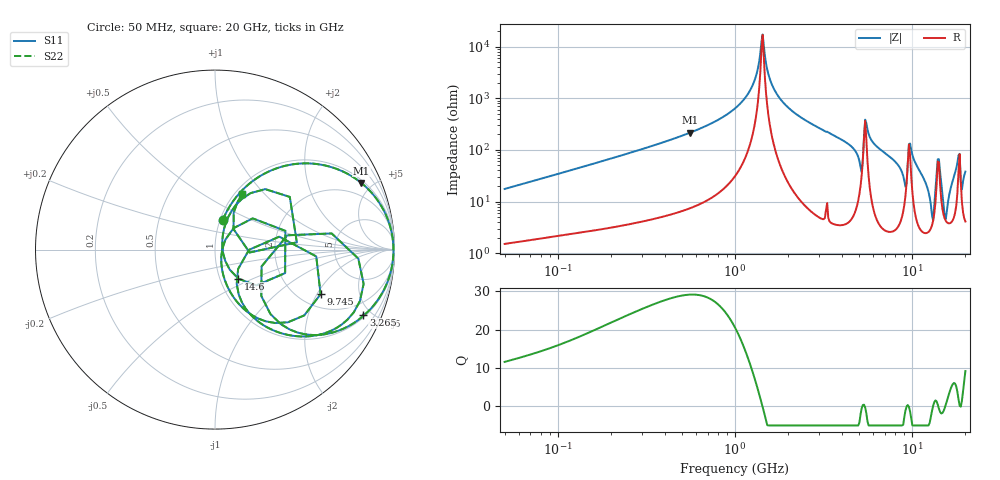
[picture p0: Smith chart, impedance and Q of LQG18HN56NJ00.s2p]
!Murata Part Number: LQG18HN56NJ00
!These Parameters are Measured in Series Mode Connection
!  o--[Z]--o
!Port1  Port2
!  o-------o
!Freq. Start=50[MHz] Stop=20[GHz], 401[Steps]
# Hz S RI R 50
!Freq.(Hz) S11(Real) S11(Imag) S21(Real) S21(Imag) S12(Real) S12(Imag) S22(Real) S22(Imag)
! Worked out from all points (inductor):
!   401 points, 50 MHz to 20 GHz, reference 50 ohm
!   read as one part in series: L = 54.9 nH near 51.52 MHz
!   highest Q = 29.1 at 557.6 MHz (marker M1), where L = 61.5 nH
!   self-resonance near 1.411 GHz
!   S11 on the Smith chart (normalised r, x): 50 MHz: 1.03, +0.35; 3.265 GHz: 1.14, -4.47; 9.745 GHz: 2.56, -2.15; 14.6 GHz: 1.22, -0.41; 20 GHz: 1.08, +0.76
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5e7  0.0431 0.1644  0.9569 -0.1644  0.9569 -0.1644  0.0431 0.1644
1.364002e8  0.1904 0.3664  0.8096 -0.3664  0.8096 -0.3664  0.1904 0.3664
3.721004e8  0.6303 0.4646  0.3697 -0.4646  0.3697 -0.4646  0.6303 0.4646
5.575697e8  0.8149 0.3716  0.1851 -0.3716  0.1851 -0.3716  0.8149 0.3716
1e9  0.9688 0.1511  0.0312 -0.1511  0.0312 -0.1511  0.9688 0.1511
1.251922e9  0.9906 0.0566  0.00943 -0.0566  0.00943 -0.0566  0.9906 0.0566
1.432596e9  0.9943 -0.00107  0.00567 0.00107  0.00567 0.00107  0.9943 -0.00107
1.740566e9  0.9873 -0.0856  0.0127 0.0856  0.0127 0.0856  0.9873 -0.0856
2.728004e9  0.9036 -0.2855  0.0964 0.2855  0.0964 0.2855  0.9036 -0.2855
3.265178e9  0.8258 -0.3643  0.1742 0.3643  0.1742 0.3643  0.8258 -0.3643
4.748272e9  0.4928 -0.4701  0.5072 0.4701  0.5072 0.4701  0.4928 -0.4701
5.352748e9  0.65 0.0901  0.35 -0.0901  0.35 -0.0901  0.65 0.0901
5.944466e9  0.6746 -0.4379  0.3254 0.4379  0.3254 0.4379  0.6746 -0.4379
7.442007e9  0.3623 -0.4637  0.6377 0.4637  0.6377 0.4637  0.3623 -0.4637
9.041845e9  0.121 -0.1915  0.879 0.1915  0.879 0.1915  0.121 -0.1915
9.745021e9  0.5882 -0.2485  0.4118 0.2485  0.4118 0.2485  0.5882 -0.2485
1.295331e10  0.035 -0.0397  0.965 0.0397  0.965 0.0397  0.035 -0.0397
1.396067e10  0.3918 0.1046  0.6082 -0.1046  0.6082 -0.1046  0.3918 0.1046
1.460232e10  0.1306 -0.1623  0.8694 0.1623  0.8694 0.1623  0.1306 -0.1623
1.550395e10  0.0408 0.0164  0.9592 -0.0164  0.9592 -0.0164  0.0408 0.0164
1.800918e10  0.2799 0.3369  0.7201 -0.3369  0.7201 -0.3369  0.2799 0.3369
2e10  0.1512 0.3079  0.8488 -0.3079  0.8488 -0.3079  0.1512 0.3079
